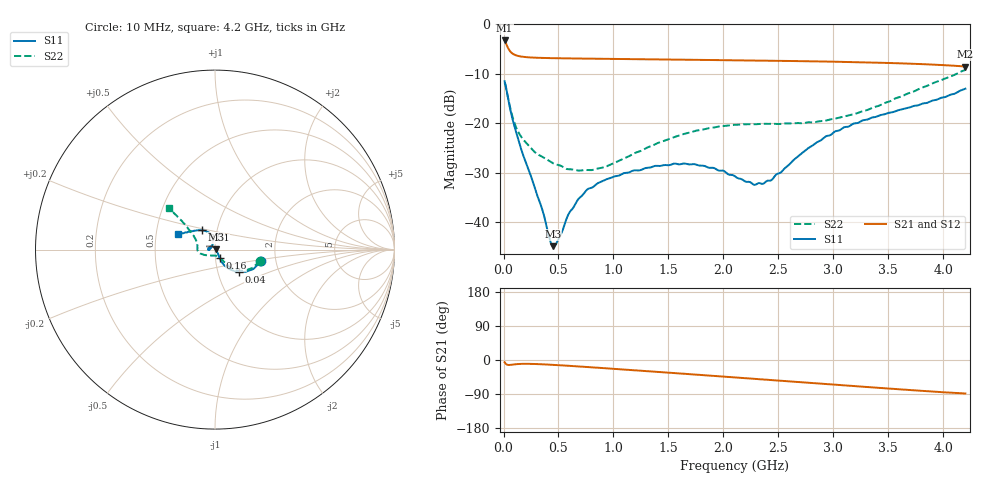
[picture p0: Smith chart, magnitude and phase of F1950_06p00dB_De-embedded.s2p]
! Integrated Device Technology
! Corporate Headquarters
! 6024 Silver Creek Valley Road
! San Jose, CA 95138  USA
! Phone:  1-408-284-8200
! Toll Free:  1-800-223-1366
! Webpage:  http://www.idt.com/
! Timing and RF Division
! 515 Groton Road, Suite 102
! Westford, MA 01886-6024
! Device:  F1950
! Description: 7-bit 0.25 dB Digital Step Attenuator
! Frequency:  150.0 -  4000.00 MHz
! Package:  4x4 mm Thin QFN Plastic Package: 24 pin
! Ports:  2 RF, 12 DC
!  Pin  1  = D0
!  Pin  2  = VDD
!  Pin  3  = Vmode
!  Pin  4  = GND
!  Pin  5  = RF1  =  Port 1
!  Pin  6  = GND
!  Pin  7  = GND
!  Pin  8  = GND
!  Pin  9  = GND
!  Pin 10  = GND
!  Pin 11  = GND
!  Pin 12  = GND
!  Pin 13  = GND
!  Pin 14  = RF2  =  Port 2
!  Pin 15  = GND
!  Pin 16  = LE
!  Pin 17  = CLK
!  Pin 18  = DATE
!  Pin 19  = D6
!  Pin 20  = D5
!  Pin 21  = D4
!  Pin 22  = D3
!  Pin 23  = D2
!  Pin 24  = D1
! State:  24
! Atten State:  6.00 dB
! Voltage:  +5.00 Volts
! Current:  Not Measured mA
! Data:  The device was measured on a the F195X evaluation board which has
!  individual transmission lines to the RF pins.  Data was collected
!  using a calibrated network analyzer.  The evaluation board was
!  de-embedded using a TRL calibration technique.
!  The reference plane is the edge of the package pin.
! Misc:  Board 2019
!  Action Tracker AT0250
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# GHz S dB R 50
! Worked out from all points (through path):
!   420 points, 10 MHz to 4.2 GHz, reference 50 ohm
!   highest |S21| = -3.27 dB at 10 MHz (marker M1); lowest = -8.5 dB at 4.2 GHz (marker M2)
!   group delay of S21, straight-line fit = 55.9 ps
!   lowest |S11| = -44.8 dB at 450 MHz (marker M3), VSWR 1.01, Z = 50.5 + j0.205 ohm
!   |S11| at or under -10 dB: start of sweep to end of sweep
!   |S22| runs from -29.6 to -9.2 dB; largest |S21 - S12| = 0.0006
!   S11 on the Smith chart (normalised r, x): 10 MHz: 1.68, -0.23; 40 MHz: 1.26, -0.33; 160 MHz: 1.05, -0.10; 3.51 GHz: 0.85, +0.19; 4.2 GHz: 0.65, +0.12
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0.01  -11.52 -13.6  -3.27 -5.9  -3.27 -5.9  -11.74 -13.7
0.04  -14.78 -43.1  -4.75 -13.0  -4.75 -13.0  -14.76 -40.6
0.1  -20.67 -60.5  -6.15 -11.5  -6.15 -11.5  -19.97 -52.1
0.16  -25.19 -61.5  -6.52 -10.3  -6.52 -10.3  -22.70 -55.5
0.29  -33.46 -51.4  -6.76 -10.6  -6.76 -10.6  -25.93 -59.6
0.36  -38.03 -35.8  -6.81 -11.4  -6.81 -11.4  -26.88 -62.7
0.42  -43.44 -7.6  -6.84 -12.3  -6.84 -12.3  -27.66 -64.5
0.45  -44.84 20.7  -6.85 -12.8  -6.85 -12.8  -28.08 -67.0
0.5  -43.43 67.5  -6.87 -13.6  -6.87 -13.6  -28.45 -70.9
0.6  -38.02 103.5  -6.90 -15.4  -6.90 -15.4  -29.31 -79.3
0.71  -34.72 117.8  -6.93 -17.5  -6.93 -17.5  -29.53 -90.1
0.93  -31.37 136.0  -6.99 -21.8  -6.99 -21.8  -28.78 -114.7
1.41  -28.63 168.7  -7.11 -31.5  -7.11 -31.6  -23.93 -151.4
1.74  -28.28 -177.4  -7.19 -38.3  -7.19 -38.4  -21.57 -164.3
2.11  -30.81 177.2  -7.29 -46.1  -7.29 -46.1  -20.34 -175.2
2.28  -32.45 154.8  -7.33 -49.6  -7.33 -49.6  -20.21 -179.6
2.37  -32.12 138.5  -7.36 -51.5  -7.36 -51.5  -20.11 178.0
2.44  -31.43 126.1  -7.38 -52.9  -7.38 -52.9  -20.10 176.0
2.81  -24.51 101.5  -7.49 -60.7  -7.49 -60.8  -19.83 163.4
3.1  -20.79 106.7  -7.60 -66.9  -7.60 -67.0  -18.65 154.3
3.51  -17.86 123.1  -7.83 -75.5  -7.82 -75.6  -15.60 143.8
4.2  -13.02 157.0  -8.54 -88.4  -8.54 -88.4  -9.21 138.0
